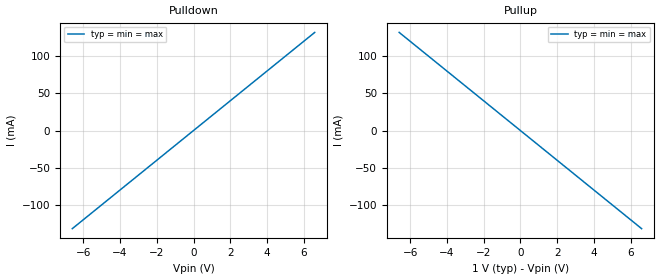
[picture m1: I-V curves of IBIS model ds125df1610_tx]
|Texas Instruments Incorporated
|16 channel retimer with integrated signal conditioning which includes
|an input Continuous-Time Linear Equalizer (CTLE),
|clock and data recovery (CDR)
|and transmit driver on each channel.
| Marketing part#   Voltage Range   Package-type   #pins
| D125DF1610   +2.375 to +2.625   FCBGA   196
[IBIS Ver]   5.1
[File Name]   ds125df1610_tx.ibs
[File Rev]   1.0
[Component]   ds125df1610_tx
[Manufacturer] Texas Instruments
[Disclaimer]
 This product is designed as an aid for customers of Texas Instruments.
 No warranties, either expressed or implied, with respect to this third
 party software (if any) or with respect to its fitness for any
 particular purpose is claimed by Texas Instruments or the author. The
 software (if any) is provided solely on an "as is" basis. The entire
 risk as to its quality and performance is with the customer
[Copyright] (C) Copyright 2017 Texas Instruments Incorporated.
   All rights reserved.
[Package]
R_pkg  0.0   NA   NA
L_pkg  0.0   NA   NA
C_pkg  0.0   NA   NA
[Pin]   signal_name   model_name   R_pin L_pin  C_pin
1p   ds125df1610_tx_p   ds125df1610_tx
1n   ds125df1610_tx_n   ds125df1610_tx
[Diff_Pin] inv_pin vdiff tdelay_typ tdelay_min tdelay_max
1p   1n   NA   NA   NA   NA
| Models and submodels in the file (1): ds125df1610_tx (Output)
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[Model] ds125df1610_tx
Model_type Output
C_comp 0p 0p 0p
Cref = 0
Vref = 0.5
Rref = 50
Vmeas = 0.5
[Temperature_Range] 25 125 0
[Voltage Range] 1.0 1.0 1.0
[Algorithmic Model]
Executable Windows_cl17.00.50727.1_64 ds125df1610_tx_x64.dll ds125df1610_tx.ami
Executable Windows_cl17.00.50727.1_32 ds125df1610_tx.dll ds125df1610_tx.ami
[End Algorithmic Model]
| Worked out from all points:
|   slope of the pulldown table from 0 to 0.15 V, typ, clamps not added: 50 ohm
|   slope of the pullup table from 0 to 0.15 V, typ, clamps not added: 50 ohm
[Pulldown]
-6.6V     -132mA     -132mA     -132mA
0V        0A         0A         0A
6.6V      132mA      132mA      132mA
[Pullup]
-6.6V     132mA      132mA      132mA
0V        0A         0A         0A
6.6V      -132mA     -132mA     -132mA
[GND Clamp]
-6.6V     0A         0A         0A
0V        0A         0A         0A
6.6V      0A         0A         0A
[Power Clamp]
-6.6V     0A         0A         0A
0V        0A         0A         0A
6.6V      0A         0A         0A
[Ramp]
dV/dt_r 0.3/1.5p 0.3/1.5p 0.3/1.5p
dV/dt_f 0.3/1.5p 0.3/1.5p 0.3/1.5p
